| IBIS file stm32wl_e5_e4_55_54_ufbga73.ibs
[IBIS ver]   4.2
[File name]  stm32wl_e5_e4_55_54_ufbga73.ibs
[File Rev]   1.0
[Date]   20-12-2019
[Source]   Data Created at STMicroelectronics
[Notes]   File originated from ELDO simulations.
[Disclaimer] This information is for modeling purpose only and is
   not guaranted. The information is subject to change without
   notice.
[Copyright]  Copyright 2019 STMicroelectronics Inc.
|   Component stm32wl_e5_e4_55_54_ufbga73
[Component] stm32wl_e5_e4_55_54_ufbga73
[Manufacturer] STMicroelectronics
[Package]
| variable   typ   min   max
R_pkg   0   NA   NA
L_pkg   0   NA   NA
C_pkg   0   NA   NA
[Pin]   signal_name   model_name   R_pin   L_pin   C_pin   | Comment
A1 VSSSMPS GND
A2 VDDSMPS POWER
A4 PA14 io8prog2m25m50m120m_sudq_ft
A5 VDDA POWER
A7 VDD POWER
A8 VBAT POWER
A9 PA12 io8prog2m25m50m120m_sudq_i2c_ft
B1 VLXSMPS POWER
B2 VFBSMPS POWER
B3 PA15 io8prog2m25m50m120m_sudq_i2c_ft
B4 PB15 io8prog2m25m50m120m_sudq_i2c_ft
B5 VREFP NC
B6 PC14 io8prog2m25m50m120m_sudq_ft
B7 VSS GND
B8 PA13 io8prog2m25m50m120m_sudq_ft
B9 PA11 io8prog2m25m50m120m_sudq_i2c_ft
C1 PB3 io8prog2m25m50m120m_sudq_ft
C2 PB4 io8prog2m25m50m120m_sudq_i2c_ft
C3 PB7 io8prog2m25m50m120m_sudq_i2c_ft
C4 PB9 io8prog2m25m50m120m_sudq_i2c_ft
C5 PC15 io8prog2m25m50m120m_sudq_ft
C6 PB14 io8prog2m25m50m120m_sudq_i2c_ft
C7 PC13 io8prog2m25m50m120m_sudq_ft
C8 PA10 io8prog2m25m50m120m_sudq_i2c_ft
D2 PB5 io8prog2m25m50m120m_sudq_ft
D3 PB8 io8prog2m25m50m120m_sudq_i2c_ft
D4 PC2 io8prog2m25m50m120m_sudq_ft
D5 PC3 io8prog2m25m50m120m_sudq_ft
D6 PA0 io8prog2m25m50m120m_sudq_ft
D7 PB13 io8prog2m25m50m120m_sudq_i2c_ft
D8 PB2 io8prog2m25m50m120m_sudq_ft
D9 VSS GND
E1 PB6 io8prog2m25m50m120m_sudq_i2c_ft
E2 VDD POWER
E3 VSS GND
E4 PC5 io8prog2m25m50m120m_sudq_ft
E5 PA9 io8prog2m25m50m120m_sudq_i2c_ft
E6 PB12 io8prog2m25m50m120m_sudq_ft
E7 PB1 io8prog2m25m50m120m_sudq_ft
E8 VDDRF POWER
E9 VDD POWER
F1 PC1 io8prog2m25m50m120m_sudq_i2c_ft
F2 PC0 io8prog2m25m50m120m_sudq_i2c_ft
F3 PC4 io8prog2m25m50m120m_sudq_ft
F4 PA6 io8prog2m25m50m120m_sudq_ft
F5 NRST ioreset_ft_v33
F6 PB0 io8prog2m25m50m120m_sudq_ft
F7 VDDRF1V55 POWER
F8 OSC-OUT NC
G2 PC6 io8prog2m25m50m120m_sudq_ft
G3 PA1 io8prog2m25m50m120m_sudq_ft
G4 PB11 io8prog2m25m50m120m_sudq_i2c_ft
G5 VSS GND
G6 VSSRF GND
G7 VSSRF GND
G8 VSSRF GND
G9 OSC-IN NC
H1 PA3 io8prog2m25m50m120m_sudq_ft
H2 PA2 io8prog2m25m50m120m_sudq_ft
H3 PA7 io8prog2m25m50m120m_sudq_i2c_ft
H4 PB10 io8prog2m25m50m120m_sudq_i2c_ft
H5 VDD POWER
H6 VSSRF GND
H7 RFI_N NC
H8 VDDPA POWER
H9 VR_PA NC
J1 PA4 io8prog2m25m50m120m_sudq_ft
J2 PA5 io8prog2m25m50m120m_sudq_ft
J3 PA8 io8prog2m25m50m120m_sudq_ft
J5 PH3 io8prog2m25m50m120m_sudq_ft
J6 RFI_P NC
J8 RFO_LP NC
J9 RFO_HP NC
[Model Selector] io8prog2m25m50m120m_sudq_ft
iols8p_sudq_ft_pd_lv  "IO low speed, PD=40kOhm - 1P8V"
iols8p_sudq_ft_pu_lv  "IO low speed, PU=40kOhm - 1P8V"
iols8p_sudq_ft_lv  "IO low speed - 1P8V"
iols8p_sudq_ft_pd  "IO low speed, PD=40kOhm - 3P3V"
iols8p_sudq_ft_pu  "IO low speed, PU=40kOhm - 3P3V"
iols8p_sudq_ft  "IO low speed - 3P3V"
iofs8p_sudq_ft_pd_lv  "IO full speed, PD=40kOhm - 1P8V"
iofs8p_sudq_ft_pu_lv  "IO full speed, PU=40kOhm - 1P8V"
iofs8p_sudq_ft_lv  "IO full speed - 1P8V"
iofs8p_sudq_ft_pd  "IO full speed, PD=40kOhm - 3P3V"
iofs8p_sudq_ft_pu  "IO full speed, PU=40kOhm - 3P3V"
iofs8p_sudq_ft  "IO full speed - 3P3V"
ioms8p_sudq_ft_pd_lv  "IO medium speed, PD=40kOhm - 1P8V"
ioms8p_sudq_ft_pu_lv  "IO medium speed, PU=40kOhm - 1P8V"
ioms8p_sudq_ft_lv  "IO medium speed - 1P8V"
ioms8p_sudq_ft_pd  "IO medium speed, PD=40kOhm - 3P3V"
ioms8p_sudq_ft_pu  "IO medium speed, PU=40kOhm - 3P3V"
ioms8p_sudq_ft  "IO medium speed - 3P3V"
iohs8p_sudq_ft_pd_lv  "IO high speed, PD=40kOhm - 1P8V"
iohs8p_sudq_ft_pu_lv  "IO high speed, PU=40kOhm - 1P8V"
iohs8p_sudq_ft_lv  "IO high speed - 1P8V"
iohs8p_sudq_ft_pd  "IO high speed, PD=40kOhm - 3P3V"
iohs8p_sudq_ft_pu  "IO high speed, PU=40kOhm - 3P3V"
iohs8p_sudq_ft  "IO high speed - 3P3V"
[Model Selector] io8prog2m25m50m120m_sudq_i2c_ft
io8prog_1v8_i2c_pd  "5V Tol GPIO 1.8V range i2c functionality with pull down"
io8prog_1v8_i2c_pu  "5V Tol GPIO 1.8V range i2c functionality with pull up"
io8prog_1v8_i2c  "5V Tol GPIO 1.8V range i2c functionality"
io8prog_3v3_i2c_pd  "5V Tol GPIO 3.3V range i2c functionality with pull down"
io8prog_3v3_i2c_pu  "5V Tol GPIO 3.3V range i2c functionality with pull up"
io8prog_3v3_i2c  "5V Tol GPIO 3.3V range i2c functionality"
io8ls_1v8_pd  "5V Tol GPIO 1.8V range with pd io low speed"
io8ls_1v8_pu  "5V Tol GPIO 1.8V range with pu io low speed"
io8ls_1v8  "5V Tol GPIO 1.8V range io low speed"
io8ls_3v3_pd  "5V Tol GPIO 3.3V range with pd io low speed"
io8ls_3v3_pu  "5V Tol GPIO 3.3V range with pu io low speed"
io8ls_3v3  "5V Tol GPIO 3.3V range io low speed"
io8fs_1v8_pd  "5V Tol GPIO 1.8V range with pd io full speed"
io8fs_1v8_pu  "5V Tol GPIO 1.8V range with pu io full speed"
io8fs_1v8  "5V Tol GPIO 1.8V range io full speed"
io8fs_3v3_pd  "5V Tol GPIO 3.3V range with pd io full speed"
io8fs_3v3_pu  "5V Tol GPIO 3.3V range with pu io full speed"
io8fs_3v3  "5V Tol GPIO 3.3V range io full speed"
io8ms_1v8_pd  "5V Tol GPIO 1.8V range with pd io medium speed"
io8ms_1v8_pu  "5V Tol GPIO 1.8V range with pu io medium speed"
io8ms_1v8  "5V Tol GPIO 1.8V range io medium speed"
io8ms_3v3_pd  "5V Tol GPIO 3.3V range with pd io medium speed"
io8ms_3v3_pu  "5V Tol GPIO 3.3V range with pu io medium speed"
io8ms_3v3  "5V Tol GPIO 3.3V range io medium speed"
io8hs_1v8_pd  "5V Tol GPIO 1.8V range with pd io high speed"
io8hs_1v8_pu  "5V Tol GPIO 1.8V range with pu io high speed"
io8hs_1v8  "5V Tol GPIO 1.8V range io high speed"
io8hs_3v3_pd  "5V Tol GPIO 3.3V range with pd io high speed"
io8hs_3v3_pu  "5V Tol GPIO 3.3V range with pu io high speed"
io8hs_3v3  "5V Tol GPIO 3.3V range io high speed"
[Model Selector] ioreset_ft_v33
ioreset_1v2_pu  "RESET 1.2V range with PU"
ioreset_1v2  "RESET 1.2V range"
ioreset_1v8_pu  "RESET 1.8V range with PU"
ioreset_1v8  "RESET 1.8V range"
ioreset_3v3_pu  "RESET 3.3V range with PU"
ioreset_3v3  "RESET 3.3V range"
| Models and submodels in the file (60): iols8p_sudq_ft_pd_lv (I/O), iols8p_sudq_ft_pu_lv (I/O), iols8p_sudq_ft_lv (I/O), iols8p_sudq_ft_pd (I/O), iols8p_sudq_ft_pu (I/O), iols8p_sudq_ft (I/O), iofs8p_sudq_ft_pd_lv (I/O), iofs8p_sudq_ft_pu_lv (I/O), iofs8p_sudq_ft_lv (I/O), iofs8p_sudq_ft_pd (I/O), iofs8p_sudq_ft_pu (I/O), iofs8p_sudq_ft (I/O), ioms8p_sudq_ft_pd_lv (I/O), ioms8p_sudq_ft_pu_lv (I/O), ioms8p_sudq_ft_lv (I/O), ioms8p_sudq_ft_pd (I/O), ioms8p_sudq_ft_pu (I/O), ioms8p_sudq_ft (I/O), iohs8p_sudq_ft_pd_lv (I/O), iohs8p_sudq_ft_pu_lv (I/O), iohs8p_sudq_ft_lv (I/O), iohs8p_sudq_ft_pd (I/O), iohs8p_sudq_ft_pu (I/O), iohs8p_sudq_ft (I/O), io8prog_1v8_i2c_pd (I/O), io8prog_1v8_i2c_pu (I/O), io8prog_1v8_i2c (I/O), io8prog_3v3_i2c_pd (I/O), io8prog_3v3_i2c_pu (I/O), io8prog_3v3_i2c (I/O), io8ls_1v8_pd (I/O), io8ls_1v8_pu (I/O), io8ls_1v8 (I/O), io8ls_3v3_pd (I/O), io8ls_3v3_pu (I/O), io8ls_3v3 (I/O), io8fs_1v8_pd (I/O), io8fs_1v8_pu (I/O), io8fs_1v8 (I/O), io8fs_3v3_pd (I/O), io8fs_3v3_pu (I/O), io8fs_3v3 (I/O), io8ms_1v8_pd (I/O), io8ms_1v8_pu (I/O), io8ms_1v8 (I/O), io8ms_3v3_pd (I/O), io8ms_3v3_pu (I/O), io8ms_3v3 (I/O), io8hs_1v8_pd (I/O), io8hs_1v8_pu (I/O), io8hs_1v8 (I/O), io8hs_3v3_pd (I/O), io8hs_3v3_pu (I/O), io8hs_3v3 (I/O), ioreset_1v2_pu (I/O_open_drain), ioreset_1v2 (I/O_open_drain), ioreset_1v8_pu (I/O_open_drain), ioreset_1v8 (I/O_open_drain), ioreset_3v3_pu (I/O_open_drain), ioreset_3v3 (I/O_open_drain)
